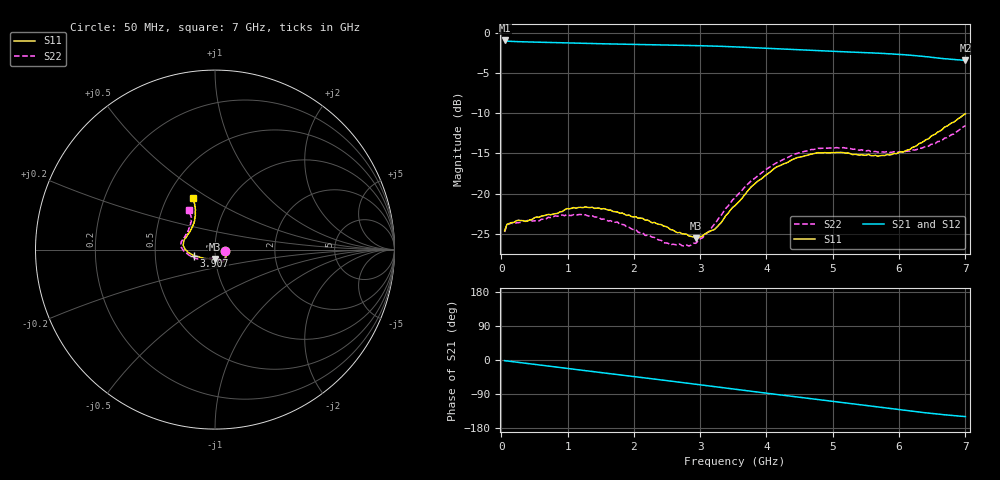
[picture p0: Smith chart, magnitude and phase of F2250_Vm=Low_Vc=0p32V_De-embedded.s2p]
! Integrated Device Technology
! Corporate Headquarters
! 6024 Silver Creek Valley Road
! San Jose, CA 95138  USA
! Phone:  1-408-284-8200
! Toll Free:  1-800-223-1366
! Webpage:  http://www.idt.com/
! Timing and RF Division
! 515 Groton Road, Suite 102
! Westford, MA 01886-6024
! Device:  F2250
! Description: Voltage Variable RF Attenuator
! Frequency:  50.0 -  6000.00 MHz
! Package:  3x3 mm Thin QFN Plastic Package: 16 pin
! Ports:  2 RF, 3 DC
!  Pin  1  = GND
!  Pin  2  = NC
!  Pin  3  = RF1  = Port 1
!  Pin  4  = NC
!  Pin  5  = GND
!  Pin  6  = GND
!  Pin  7  = GND
!  Pin  8  = GND
!  Pin  9  = NC
!  Pin 10  = RF2  = Port 2
!  Pin 11  = NC
!  Pin 12  = GND
!  Pin 13  = GND
!  Pin 14  = VCNTRL
!  Pin 15  = VDD
!  Pin 16  = VMODE
! Vcntrl:  0.320 Volts
! Vmode:  +0.000 Volts
! Vdd:  +3.30  Volts
! Current:  1.116 mA
! Data:  The device was measured on a the F2250 evaluation board which has
!  individual transmission lines to the RF pins.  Data was collected
!  using a calibrated network analyzer.  The evaluation board was
!  de-embedded using a TRL calibration technique.
!  The reference plane is the edge of the package pin.
! Misc:  SN 10
!  Action Tracker AT0258
! Date Measured:  2014-11-26
! Date:  2015-10-15  MJV
! Note:
!  Integrated Device Technology supplies this data as a sample of measured
!  data at the package pin for this product.  Your particular data for this
!  product may vary.
!  Data was taken at 25 degrees C.
!  Integrated Device Technology reserves the right to change this data at anytime.
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# GHz S dB R 50
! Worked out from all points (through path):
!   201 points, 50 MHz to 7 GHz, reference 50 ohm
!   highest |S21| = -0.96 dB at 50 MHz (marker M1); lowest = -3.4 dB at 7 GHz (marker M2)
!   group delay of S21, straight-line fit = 60 ps
!   lowest |S11| = -25.6 dB at 2.934 GHz (marker M3), VSWR 1.11, Z = 49.7 - j5.26 ohm
!   |S11| at or under -10 dB: start of sweep to end of sweep
!   |S22| runs from -26.5 to -11.5 dB; largest |S21 - S12| = 0.00031
!   S11 on the Smith chart (normalised r, x): 50 MHz: 1.12, -0.02; 3.907 GHz: 0.79, -0.05; 7 GHz: 0.67, +0.43
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0.05  -24.63 -9.3  -0.96 -1.8  -0.96 -1.8  -24.77 -9.8
0.08475  -23.82 -9.2  -1.03 -2.5  -1.03 -2.5  -23.89 -9.1
0.15425  -23.60 -11.4  -1.07 -4.0  -1.07 -4.0  -23.67 -10.8
0.57125  -22.93 -29.0  -1.18 -13.1  -1.17 -13.1  -23.39 -29.9
0.884  -22.26 -44.5  -1.24 -19.9  -1.24 -19.9  -22.68 -46.1
1.2315  -21.74 -54.5  -1.32 -27.4  -1.31 -27.4  -22.68 -58.9
1.75275  -22.28 -61.3  -1.41 -38.4  -1.41 -38.4  -23.52 -66.2
2.37825  -23.82 -62.2  -1.50 -51.8  -1.50 -51.8  -25.76 -68.4
2.552  -24.47 -66.2  -1.52 -55.6  -1.52 -55.6  -26.39 -74.1
2.83  -25.27 -81.0  -1.58 -61.7  -1.57 -61.7  -26.52 -92.8
2.93425  -25.56 -89.8  -1.60 -64.0  -1.59 -64.0  -26.17 -101.4
3.21225  -24.47 -119.0  -1.66 -70.2  -1.66 -70.2  -23.82 -126.8
3.525  -21.50 -146.1  -1.75 -77.1  -1.76 -77.1  -20.51 -145.7
3.76825  -19.16 -159.7  -1.85 -82.5  -1.85 -82.5  -18.41 -156.2
3.90725  -18.25 -164.1  -1.90 -85.5  -1.90 -85.5  -17.53 -162.4
4.1505  -16.69 -172.6  -2.00 -90.8  -2.00 -90.8  -16.17 -171.0
4.7065  -15.04 173.1  -2.21 -102.9  -2.21 -102.9  -14.51 175.9
5.15825  -14.90 162.4  -2.37 -112.6  -2.37 -112.6  -14.28 166.7
5.85325  -15.19 139.1  -2.62 -127.5  -2.62 -127.5  -14.89 151.5
6.166  -14.50 128.2  -2.78 -134.3  -2.79 -134.4  -14.71 142.7
6.444  -13.19 119.8  -2.99 -140.1  -3.00 -140.1  -14.10 133.3
7  -10.08 113.4  -3.44 -149.4  -3.44 -149.4  -11.55 123.8
